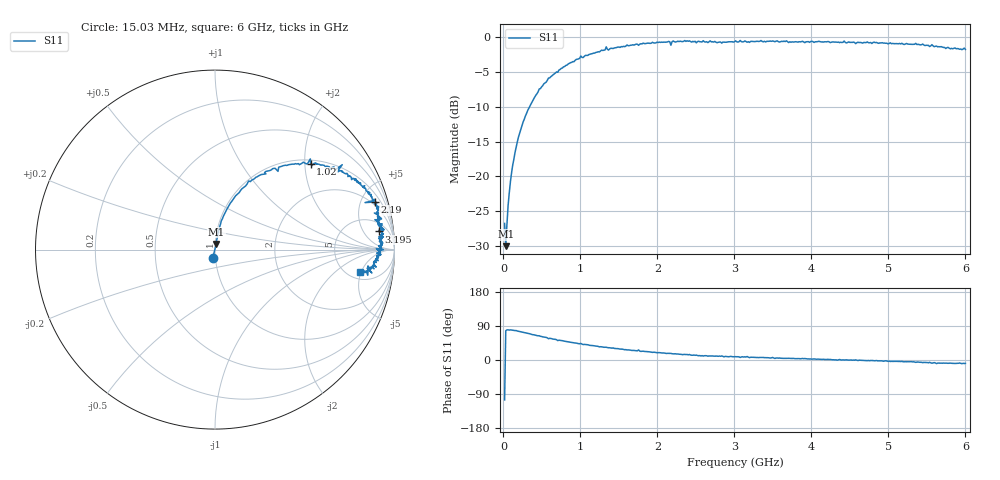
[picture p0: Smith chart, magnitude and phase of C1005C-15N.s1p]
!	Network	Analyzer	HP8753E.07.74:	Oct	30	2002	Serial	No.	JP38451487
!	Hewlett-Packard
!	7	Sep	2009	8:46:56
!	Frequency	S11
#	HZ	S	RI	R	50
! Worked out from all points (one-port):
!   400 points, 15.03 MHz to 6 GHz, reference 50 ohm
!   lowest |S11| = -30.0 dB at 30.03 MHz (marker M1), VSWR 1.07, Z = 50.6 + j3.12 ohm
!   |S11| at or under -10 dB: start of sweep to 338.7 MHz
!   S11 on the Smith chart (normalised r, x): 15.03 MHz: 0.97, -0.09; 1.02 GHz: 1.09, +2.14; 2.19 GHz: 1.69, +6.42; 3.195 GHz: 9, +11; 6 GHz: 6.25, -4.79
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1.502992e7  -0.0121 -0.0444
3.002985e7  0.00701 0.0308
6.00297e7  0.011 0.0605
1.050295e8  0.0202 0.104
1.650292e8  0.0346 0.159
2.550287e8  0.072 0.235
4.650277e8  0.187 0.382
7.650262e8  0.378 0.467
1.020025e9  0.533 0.479
1.335023e9  0.709 0.473
1.515022e9  0.74 0.407
1.725021e9  0.811 0.371
1.755021e9  0.782 0.392
1.93502e9  0.863 0.317
2.145019e9  0.89 0.279
2.175019e9  0.836 0.262
2.190019e9  0.889 0.265
2.265019e9  0.9 0.256
2.565017e9  0.91 0.172
3.015015e9  0.931 0.144
3.075015e9  0.941 0.111
3.165014e9  0.908 0.147
3.195014e9  0.912 0.101
3.765011e9  0.92 0.0697
4.515007e9  0.919 0.000854
5.265004e9  0.888 -0.0712
5.625002e9  0.851 -0.143
6e9  0.808 -0.127
